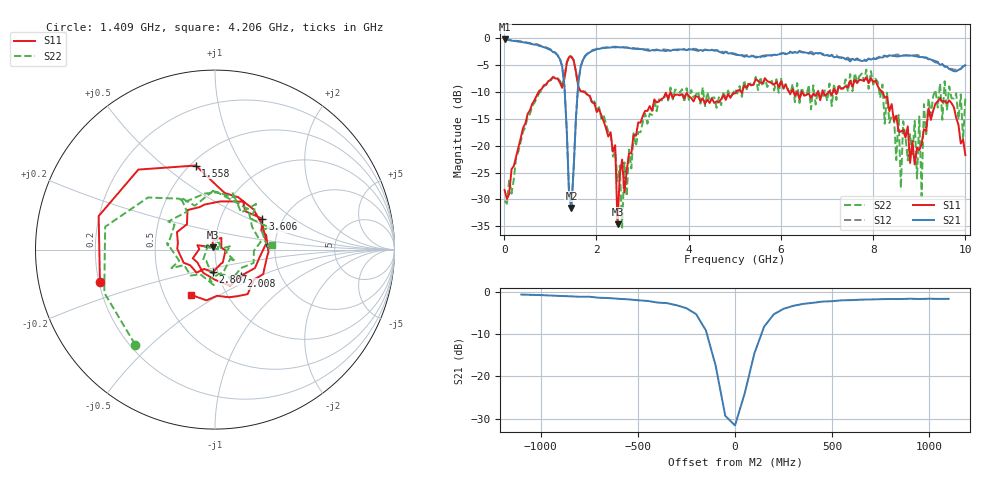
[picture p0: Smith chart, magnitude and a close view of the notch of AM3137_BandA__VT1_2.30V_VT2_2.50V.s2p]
! Date/Time: Tue, Nov 13, 2018 4:48 PM
! Network Analyzer: Agilent Technologies E8364B Rev: A.07.50.67
! Sweep from 0.010 to 10.000 GHz, 201 Points, Sweep Type: LIN
! Power Supply: 2.301 V, -0.000 A
# Hz S DB R 50
!freq MagS11 AngS11 MagS21 AngS21 MagS12 AngS12 MagS22 AngS22
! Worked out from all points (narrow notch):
!   201 points, 10 MHz to 10 GHz, reference 50 ohm
!   highest |S21| = -0.26 dB at 10 MHz (marker M1); lowest = -31.6 dB at 1.459 GHz (marker M2)
!   notch at M2: 28.6 dB deep, 187 MHz wide at half that depth
!   lowest |S11| = -34.6 dB at 2.458 GHz (marker M3), VSWR 1.04, Z = 48.6 + j1.21 ohm
!   |S11| at or under -10 dB: start of sweep to 748.6 MHz; 1.725 GHz to 5.034 GHz (3.309 GHz wide, 97.9 % of centre); 8.202 GHz to end of sweep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
!   |S22| runs from -35.3 to -3.2 dB; largest |S21 - S12| = 0.028
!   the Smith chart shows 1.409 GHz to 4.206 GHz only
!   S11 on the Smith chart (normalised r, x): 1.409 GHz: 0.20, -0.13; 1.558 GHz: 0.53, +0.65; 2.008 GHz: 1.27, -0.39; 2.807 GHz: 0.95, -0.24; 3.606 GHz: 1.58, +0.60; 4.206 GHz: 0.68, -0.37
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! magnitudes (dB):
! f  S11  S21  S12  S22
! 10 MHz  -28.2  -0.3  -0.2  -30.2
! 1.209 GHz  -8.3  -3.9  -3.9  -8.0
! 1.409 GHz  -3.5  -29.3  -29.2  -3.2
! 1.459 GHz  -3.4  -31.6  -31.4  -3.6
! 1.558 GHz  -6.4  -14.6  -14.5  -6.5
! 1.708 GHz  -9.9  -4.1  -4.0  -10.0
! 2.008 GHz  -13.8  -2.1  -2.0  -13.3
! 2.408 GHz  -19.9  -1.8  -1.6  -21.1
! 2.458 GHz  -34.6  -1.7  -1.7  -26.6
! 2.807 GHz  -18.0  -2.0  -1.9  -17.7
! 3.357 GHz  -11.8  -2.3  -2.2  -11.4
! 3.606 GHz  -10.0  -2.4  -2.4  -9.2
! 4.206 GHz  -10.9  -2.4  -2.2  -9.9
! 5.005 GHz  -10.3  -3.1  -2.9  -9.4
! 6.703 GHz  -10.3  -3.1  -2.8  -8.8
! 8.352 GHz  -13.6  -3.2  -3.3  -15.8
! 8.551 GHz  -17.3  -3.4  -3.1  -14.3
! 8.601 GHz  -17.4  -3.3  -3.1  -27.9
! 9.001 GHz  -20.8  -3.5  -3.3  -14.6
! 9.051 GHz  -19.7  -3.5  -3.3  -29.4
! 9.101 GHz  -17.0  -3.6  -3.6  -12.3
! 10 GHz  -21.8  -5.1  -5.0  -10.9
